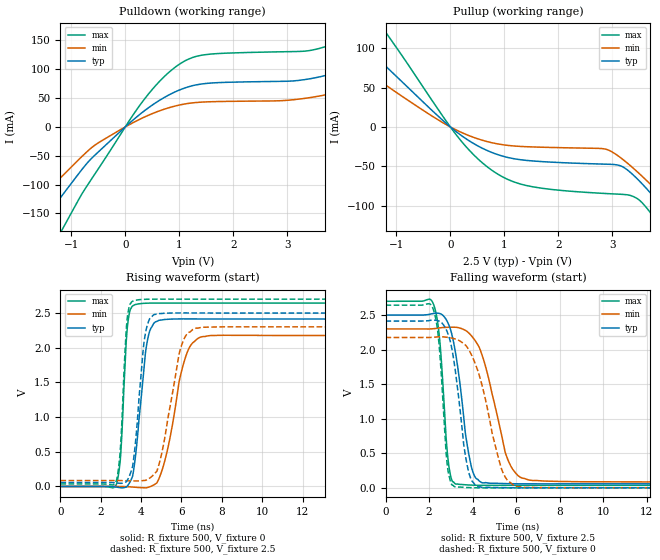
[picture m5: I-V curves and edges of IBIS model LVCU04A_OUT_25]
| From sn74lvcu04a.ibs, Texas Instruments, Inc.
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[Model]   LVCU04A_OUT_25
Model_type  Output
Vref =   0
Rref =   500
Cref =   30p
Vmeas =   1.25
| variable   typ   min   max
C_comp   8.09pF   4.04pF   13.68pF
| C_pullup   6.98pF   4.04pF   8.26pF
| C_pulldown   9.19pF   4.38pF   13.68pF
[Temperature Range]   40   100   -40
| Ambient temperature   25   85   -40
[Voltage range]   2.5   2.3   2.7
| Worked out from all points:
|   slope of the pulldown table from 0 to 0.375 V, typ, clamps not added: 12.7 ohm
|   slope of the pullup table from 0 to 0.375 V, typ, clamps not added: 20 ohm
|   rising waveform, R_fixture 500, V_fixture 0: 20-80 % time 477ps typ, 845ps min, 267ps max; typ from 0 V to 2.41 V
|   falling waveform, R_fixture 500, V_fixture 2.5: 20-80 % time 610ps typ, 987ps min, 343ps max; typ from 2.5 V to 0.057 V
|   rising waveform, R_fixture 500, V_fixture 2.5: 20-80 % time 428ps typ, 793ps min, 266ps max; typ from 0.057 V to 2.5 V
|   falling waveform, R_fixture 500, V_fixture 0: 20-80 % time 569ps typ, 998ps min, 331ps max; typ from 2.41 V to 0 V
[Pulldown]
| LVCU04A_OUT_25
|   Voltage   I(typ)   I(min)   I(max)
-5.5V     -601.9mA   -483.7mA   -770.2mA
-2.12V    -234.1mA   -175.5mA   -328.1mA
-1.58V    -169.3mA   -124.4mA   -246.1mA
-1.15V    -116.5mA   -83.59mA   -175.1mA
-565mV    -49.19mA   -31.73mA   -81.94mA
365mV     28.75mA    17.58mA    49.46mA
1.32V     73.05mA    42.4mA     122.5mA
4V        96.78mA    61.72mA    149.2mA
4.6V      117.3mA    77.78mA    177.9mA
5.77V     171.8mA    120.4mA    253.2mA
7.055V    245.3mA    179.5mA    351.5mA
11V       504.9mA    394.6mA    686.5mA
[Pullup]
| LVCU04A_OUT_25
|   Voltage   I(typ)   I(min)   I(max)
-5.5V     363.4mA    279.9mA    508.8mA
-2.6V     169.4mA    122.6mA    251.6mA
-1.815V   117.7mA    83.03mA    179.1mA
-1.37V    88.47mA    61.37mA    136.9mA
170mV     -9.222mA   -5.867mA   -15.32mA
760mV     -32.2mA    -19.89mA   -54.58mA
2.88V     -47.3mA    -28.27mA   -84.56mA
3.45V     -65.22mA   -56.26mA   -90.57mA
3.915V    -100.8mA   -87.46mA   -129mA
4.185V    -124.1mA   -107.2mA   -157.5mA
4.495V    -152.3mA   -130.9mA   -192.5mA
11V       -836.4mA   -705.6mA   -1.028A
[Ramp]
| LVCU04A_OUT_25
| variable   typ   min   max
dV/dt_r   1.46/5.15E-10   1.32/9.18E-10   1.60/2.82E-10
dV/dt_f   1.48/6.59E-10   1.34/1.04E-09   1.62/3.68E-10
R_load = 500
[Rising Waveform]
| LVCU04A_OUT_25
R_fixture =   500
C_fixture =   0
L_fixture =   0
V_fixture =   0
V_fixture_min = 0
V_fixture_max = 0
|   Time   V(typ)   V(min)   V(max)
0s        177.7pV    3.876nV    17.91pV
2.78ns    -9.713mV   402uV      34.96mV
2.98ns    -18.78mV   5.148uV    435.3mV
3.325ns   9.85mV     -3.908mV   2.316V
3.7ns     388.5mV    -11.4mV    2.622V
4.28ns    2.053V     -17.72mV   2.642V
4.88ns    2.394V     110.9mV    2.644V
6.135ns   2.415V     1.803V     2.644V
6.945ns   2.414V     2.154V     2.644V
24.99ns   2.414V     2.176V     2.644V
[Falling Waveform]
| LVCU04A_OUT_25
R_fixture =   500
C_fixture =   0
L_fixture =   0
V_fixture =   2.5
V_fixture_min = 2.3
V_fixture_max = 2.7
|   Time   V(typ)   V(min)   V(max)
0s        2.5V       2.3V       2.7V
2.205ns   2.524V     2.303V     2.656V
2.495ns   2.522V     2.315V     2.121V
2.89ns    2.371V     2.324V     362.3mV
3.225ns   1.936V     2.324V     54.24mV
3.705ns   714.4mV    2.273V     43.18mV
4.09ns    170.1mV    2.143V     37.56mV
5.53ns    60.95mV    484.2mV    35.48mV
6.275ns   57.84mV    140.6mV    35.82mV
24.99ns   57.33mV    84.96mV    35.94mV
[Rising Waveform]
| LVCU04A_OUT_25
R_fixture =   500
C_fixture =   0
L_fixture =   0
V_fixture =   2.5
V_fixture_min = 2.3
V_fixture_max = 2.7
|   Time   V(typ)   V(min)   V(max)
0s        57.33mV    84.96mV    35.94mV
2.78ns    49.46mV    85.17mV    88.43mV
2.97ns    45.02mV    84.76mV    536.2mV
3.3ns     83.83mV    82.15mV    2.391V
3.66ns    472mV      79.57mV    2.68V
4.165ns   2.121V     86.76mV    2.698V
4.665ns   2.479V     181.8mV    2.7V
5.92ns    2.501V     1.953V     2.7V
6.66ns    2.501V     2.277V     2.7V
24.99ns   2.5V       2.3V       2.7V
[Falling Waveform]
| LVCU04A_OUT_25
R_fixture =   500
C_fixture =   0
L_fixture =   0
V_fixture =   0
V_fixture_min = 0
V_fixture_max = 0
|   Time   V(typ)   V(min)   V(max)
0s        2.414V     2.176V     2.644V
2.18ns    2.427V     2.179V     2.595V
2.45ns    2.414V     2.185V     2.107V
2.85ns    2.243V     2.178V     294.7mV
3.19ns    1.732V     2.155V     13.65mV
3.61ns    588.8mV    2.082V     6.596mV
3.945ns   113.9mV    1.926V     2.01mV
5.315ns   2.093mV    284.3mV    -469uV
6ns       166.7uV    21.68mV    -153.8uV
24.99ns   16.4nV     30.2nV     1.911nV
